TYPE STR_AO :
STRUCT
MFC1_Flow_Setpoint	,
MFC1_Rate_Setpoint	,
MFC2_Flow_Setpoint	,
MFC2_Rate_Setpoint	,
MFC3_Flow_Setpoint	,
MFC3_Rate_Setpoint	,
MFC4_Flow_Setpoint	,
MFC4_Rate_Setpoint	,
MFC5_Flow_Setpoint	,
MFC5_Rate_Setpoint	,
MFC6_Flow_Setpoint	,
MFC6_Rate_Setpoint	,
MFC7_Flow_Setpoint	,
MFC7_Rate_Setpoint	,
LID_Temp_SV	,	//E02
//LID_Heater2_Temperature_Setpoint	,	//E03
//LID_Heater3_Temperature_Setpoint	,	//E04
//LID_Heater4_Temperature_Setpoint	,	//E05
Chamber_Temp1_SV	,//E06
Chamber_Temp2_SV	,//E07
Chamber_Temp3_SV	,//E08
(*Chamber_Heater4_Temperature_Setpoint	,//E09
Chamber_Heater5_Temperature_Setpoint	,//E10
Chamber_Heater6_Temperature_Setpoint	,//E11
Chamber_Heater7_Temperature_Setpoint	,//E12
Chamber_Heater8_Temperature_Setpoint	,//E13*)
AV102_Temp_SV	,//E14
AV101_Temp_SV	,//E15
AV104_Temp_SV	,//E16
AV105_Temp_SV	,
//BA01_Temp_SV	,//E17
//VG103_Pipe_Temp_SV	,//E16
Exhaust1_3_Temp_SV	,//E14
Exhaust4_7_Temp_SV	,//E15
VG101_Pipe_Temp_SV	,//E16
(*Forline_Heater9_Temperature_Setpoint	,//E17
Forline_Heater10_Temperature_Setpoint	,//E14
Forline_Heater11_Temperature_Setpoint	,//E15
Forline_Heater12_Temperature_Setpoint	,//E16
Forline_Heater13_Temperature_Setpoint	,//E17
Forline_Heater14_Temperature_Setpoint	,//E14
Forline_Heater15_Temperature_Setpoint	,//E15
Forline_Heater16_Temperature_Setpoint	,//E16
Forline_Heater17_Temperature_Setpoint	,//E17
Forline_Heater18_Temperature_Setpoint	,//E14
Forline_Heater19_Temperature_Setpoint	,//E15
Forline_Heater20_Temperature_Setpoint	,//E16*)
Gate_Valve_Temp_SV	,//E18
APC_Temp_SV	,//E01
TMP_Temp_SV	,//不用
Tape_Temp1_SV	,
Tape_Temp2_SV	,
Tape_Temp3_SV	,
Tape_Temp4_SV	,
IGS_Temp1_SV	,
IGS_Temp2_SV	,
Chiller_Temp1_SV	,
Chiller_Temp2_SV	,
Stage_Temp1_SV	,
Stage_Temp2_SV	,
Stage_Temp3_SV	,
Stage_Temp4_SV	:REAL;


APC:VAT_OUT;

TMP:TMP_OUT;
END_STRUCT
END_TYPE
